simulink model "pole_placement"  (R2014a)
settings: Solver=ode45  StartTime=0.0  StopTime=10.0  RelTol=1e-3
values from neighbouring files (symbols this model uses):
  A = [0 1; 0 0]    [L9.m]    (also in L9_LandObs_script.m; L9_fullExample_script.m; L9_onlyL_script.m)
  B = [0; 1]    [L9.m]    (also in L9_LandObs_script.m; L9_fullExample_script.m; L9_onlyL_script.m)
  Cx = eye(size(A))    [L9.m]    (also in L9_LandObs_script.m; L9_fullExample_script.m; L9_onlyL_script.m)
  Dx = zeros(size(Cx,1),size(B,2))    [L9.m]    (also in L9_LandObs_script.m; L9_fullExample_script.m; L9_onlyL_script.m)
  h = h3    (= 0.5)    [L9.m]    (also in L9_LandObs_script.m = 0.44; L9_fullExample_script.m = 0.44; L9_onlyL_script.m = 0.44)
  L = L3    [L9.m]    (also in L9_LandObs_script.m = place(Phi,Gamma,pd); L9_fullExample_script.m = place(Phi,Gamma,pd); L9_onlyL_script.m = place(Phi,Gamma,pd))
  x0 = [1;1]    [L9.m]    (also in L9_LandObs_script.m; L9_fullExample_script.m; L9_onlyL_script.m)

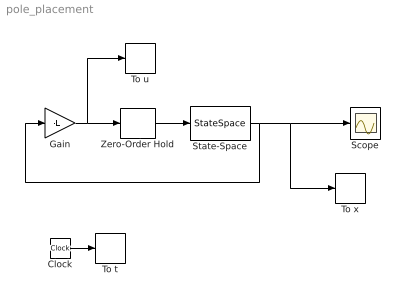
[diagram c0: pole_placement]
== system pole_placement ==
  Clock : Clock
  Gain : Gain  Gain=-L  Multiplication=Matrix(K*u)  SampleTime=h
  Scope : Scope
  State-Space : StateSpace  A=A  B=B  C=Cx  D=Dx  X0=x0
  To t : ToWorkspace  VariableName=t  SampleTime=h
  To u : ToWorkspace  VariableName=u  SampleTime=h
  To x : ToWorkspace  VariableName=x  SampleTime=h
  Zero-Order Hold : ZeroOrderHold  SampleTime=h
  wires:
  Zero-Order Hold/1 -> State-Space/1
  Gain/1 -> To u/1, Zero-Order Hold/1
  State-Space/1 -> Gain/1, To x/1, Scope/1
  Clock/1 -> To t/1
